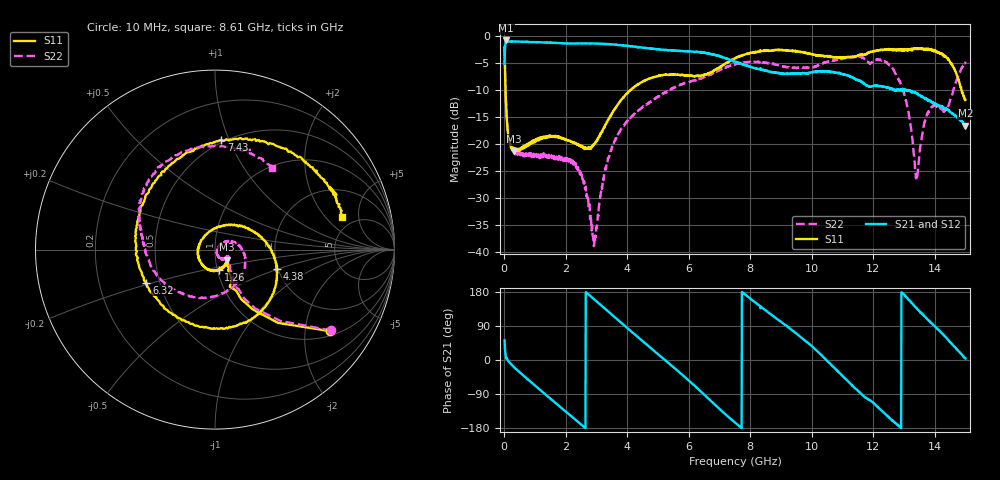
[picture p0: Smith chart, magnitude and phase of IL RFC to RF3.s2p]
!Agilent Technologies,N5230A,MY45001650,A.07.50.48
!Agilent N5230A: A.07.50.48
!Date: Wednesday, April 30, 2014 16:48:38
!Correction: S11(Full 2 Port(1,2))
!S21(Full 2 Port(1,2))
!S12(Full 2 Port(1,2))
!S22(Full 2 Port(1,2))
!S2P File: Measurements: S11, S21, S12, S22:
# Hz S  dB  R 50
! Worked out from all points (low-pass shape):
!   1500 points, 10 MHz to 15 GHz, reference 50 ohm
!   highest |S21| = -0.80 dB at 60 MHz (marker M1); lowest = -16.6 dB at 15 GHz (marker M2)
!   |S21| within 3 dB of the highest: 15.55 MHz to 7.036 GHz (7.02 GHz wide, 199 % of centre); 7.049674 GHz to 7.05031 GHz (636 kHz wide, 0.00902 % of centre)
!   lowest |S11| = -21.3 dB at 300 MHz (marker M3), VSWR 1.19, Z = 56.6 - j6.39 ohm
!   |S11| at or under -10 dB: 39.23 MHz to 4.097 GHz (4.058 GHz wide, 196 % of centre); 4.107601 GHz to 4.112062 GHz (4.461 MHz wide, 0.109 % of centre); 14.88 GHz to end of sweep
!   |S22| runs from -38.9 to -2.1 dB; largest |S21 - S12| = 0.014
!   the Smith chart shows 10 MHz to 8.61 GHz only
!   S11 on the Smith chart (normalised r, x): 10 MHz: 1.14, -2.71; 1.26 GHz: 1.02, -0.23; 4.38 GHz: 1.97, -0.49; 6.32 GHz: 0.42, -0.19; 7.43 GHz: 0.48, +0.94; 8.61 GHz: 3.95, +3.09
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1e7  -2.09 -35.3  -5.08 51.7  -5.01 51.8  -2.07 -34.9
6e7  -13.07 -68.2  -0.80 4.1  -0.84 4.0  -12.91 -62.6
3e8  -21.33 -40.8  -0.99 -17.7  -0.99 -17.7  -21.22 -31.9
1.26e9  -18.79 -79.4  -1.18 -85.6  -1.17 -85.6  -22.42 -33.8
2.51e9  -20.34 -178.4  -1.35 -171.0  -1.37 -171.0  -25.94 -61.2
2.94e9  -19.94 114.0  -1.39 159.0  -1.40 159.0  -37.42 -12.5
3.48e9  -14.55 44.8  -1.53 121.0  -1.51 121.1  -21.18 30.7
4.38e9  -8.84 -17.4  -2.07 57.9  -2.06 58.0  -13.69 -43.4
5.01e9  -7.36 -52.1  -2.45 14.7  -2.46 14.7  -11.16 -103.4
6.32e9  -7.45 -154.3  -2.95 -77.8  -3.01 -77.7  -8.01 174.6
7.43e9  -4.27 86.7  -4.52 -160.1  -4.57 -160.1  -5.33 130.2
7.51e9  -4.14 81.0  -4.74 -165.4  -4.77 -165.5  -5.17 125.6
8.61e9  -2.71 14.4  -6.55 124.0  -6.64 123.7  -5.11 55.3
1.001e10  -3.37 -66.5  -6.66 36.2  -6.71 36.0  -5.84 -44.7
1.121e10  -3.93 -179.2  -7.35 -58.7  -7.35 -58.8  -3.90 -112.8
1.192e10  -2.89 112.6  -9.34 -107.8  -9.27 -107.7  -5.03 -140.8
1.251e10  -2.46 72.5  -9.50 -151.1  -9.63 -150.9  -5.19 -168.5
1.303e10  -2.45 49.9  -9.85 169.7  -9.83 169.7  -11.11 157.7
1.341e10  -2.23 37.0  -10.53 136.5  -10.51 136.6  -26.69 55.5
1.38e10  -2.56 21.0  -11.96 104.2  -11.77 104.4  -13.92 -46.8
1.438e10  -3.90 -9.8  -13.44 58.3  -13.59 58.9  -13.46 -33.7
1.5e10  -11.84 -125.7  -16.60 3.9  -16.46 4.1  -4.73 -15.8
